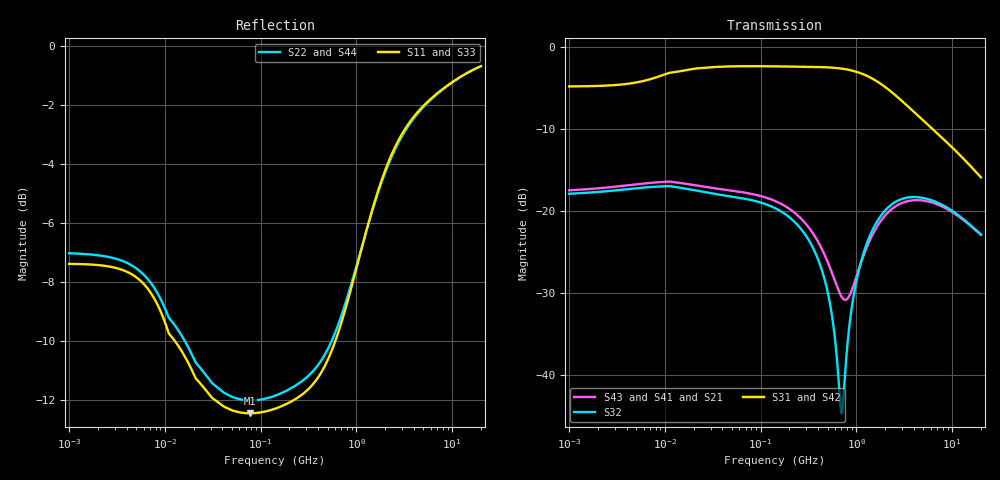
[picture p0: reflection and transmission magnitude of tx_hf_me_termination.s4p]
! Created Wed Jul 29 12:27:12 2015
# hz S db R 50
! 4 Port Network Data from SP1.SP block
! freq  dbS11  angS11  dbS12  angS12  dbS13  angS13  dbS14  angS14
!  dbS21  angS21  dbS22  angS22  dbS23  angS23  dbS24  angS24
!  dbS31  angS31  dbS32  angS32  dbS33  angS33  dbS34  angS34
!  dbS41  angS41  dbS42  angS42  dbS43  angS43  dbS44  angS44
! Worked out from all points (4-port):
!   861 points, 1 MHz to 20 GHz, reference 50 ohm
!   strongest paths, dB at 1 MHz, 11.89 MHz, 141.4 MHz, 1.682 GHz, 20 GHz:
!     S31: -4.8, -3.1, -2.4, -4.3, -15.9
!     S42: -5.1, -3.4, -2.5, -4.4, -15.9
!     S32: -17.9, -17.0, -19.7, -21.1, -22.9
!     S43: -17.5, -16.5, -18.8, -21.7, -22.9
!     S41: -17.5, -16.5, -18.8, -21.7, -22.9
!     S21: -17.5, -16.5, -18.8, -21.7, -22.9
!   lowest |S11| = -12.4 dB at 77.71 MHz (marker M1), VSWR 1.63, Z = 30.7 - j0.135 ohm
!   |S11| at or under -10 dB: 12.76 MHz to 602.8 MHz (590.1 MHz wide, 192 % of centre)
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1000000  -7.38 177.0  -17.91 1.5  -4.83 2.3  -17.91 1.5
         -17.49 1.8  -7.02 177.2  -17.49 1.8  -5.11 2.3
         -4.83 2.3  -17.91 1.5  -7.38 177.0  -17.91 1.5
         -17.49 1.8  -5.11 2.3  -17.49 1.8  -7.02 177.2
7.770567e7  -12.45 -179.5  -18.65 -18.6  -2.37 -0.2  -18.65 -18.6
            -17.89 -15.3  -12.01 -179.9  -17.89 -15.3  -2.51 -0.0
            -2.37 -0.2  -18.65 -18.6  -12.45 -179.5  -18.65 -18.6
            -17.89 -15.3  -2.51 -0.0  -17.89 -15.3  -12.01 -179.9
3.720622e8  -11.37 -159.3  -25.07 -54.3  -2.46 -7.3  -25.07 -54.3
            -23.16 -38.7  -10.93 -160.7  -23.16 -38.7  -2.64 -7.3
            -2.46 -7.3  -25.07 -54.3  -11.37 -159.3  -25.07 -54.3
            -23.16 -38.7  -2.64 -7.3  -23.16 -38.7  -10.93 -160.7
7.00941e8  -9.35 -147.5  -44.65 1.7  -2.67 -14.4  -44.65 1.7
           -30.44 -13.8  -9.12 -149.8  -30.44 -13.8  -2.86 -14.2
           -2.67 -14.4  -44.65 1.7  -9.35 -147.5  -44.65 1.7
           -30.44 -13.8  -2.86 -14.2  -30.44 -13.8  -9.12 -149.8
1.013257e9  -7.47 -144.2  -28.26 67.4  -3.07 -20.7  -28.26 67.4
            -27.84 32.0  -7.40 -146.3  -27.84 32.0  -3.26 -20.2
            -3.07 -20.7  -28.26 67.4  -7.47 -144.2  -28.26 67.4
            -27.84 32.0  -3.26 -20.2  -27.84 32.0  -7.40 -146.3
1.908911e9  -4.39 -148.4  -20.22 39.2  -4.73 -33.1  -20.22 39.2
            -20.83 28.8  -4.46 -149.4  -20.83 28.8  -4.85 -32.1
            -4.73 -33.1  -20.22 39.2  -4.39 -148.4  -20.22 39.2
            -20.83 28.8  -4.85 -32.1  -20.83 28.8  -4.46 -149.4
2e10  -0.67 -171.5  -22.87 -40.7  -15.90 -58.3  -22.87 -40.7
      -22.90 -40.6  -0.67 -171.5  -22.90 -40.6  -15.90 -58.3
      -15.90 -58.3  -22.87 -40.7  -0.67 -171.5  -22.87 -40.7
      -22.90 -40.6  -15.90 -58.3  -22.90 -40.6  -0.67 -171.5
